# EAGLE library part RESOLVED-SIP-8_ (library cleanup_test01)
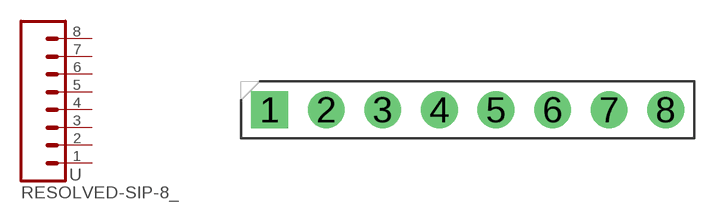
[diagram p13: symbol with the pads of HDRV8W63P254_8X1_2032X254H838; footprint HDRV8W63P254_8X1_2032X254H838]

Designator prefix -

## RESOLVED-SIP-8_2.54-SPACE-VERTICAL  [HDRV8W63P254_8X1_2032X254H838]
1  1  pas
2  2  pas
3  3  pas
4  4  pas
5  5  pas
6  6  pas
7  7  pas
8  8  pas

## Footprint HDRV8W63P254_8X1_2032X254H838 (pad centres in mm)
drill 1.1 pad 1.65 square: 1 0,0
drill 1.1 pad 1.65: 2 2.54,0; 3 5.08,0; 4 7.62,0; 5 10.16,0; 6 12.7,0; 7 15.24,0; 8 17.78,0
